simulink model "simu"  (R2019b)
settings: Solver=VariableStepAuto  StartTime=0.0  StopTime=10.0  RelTol=1e-3
libraries: fl_lib x81, nesl_utility x12

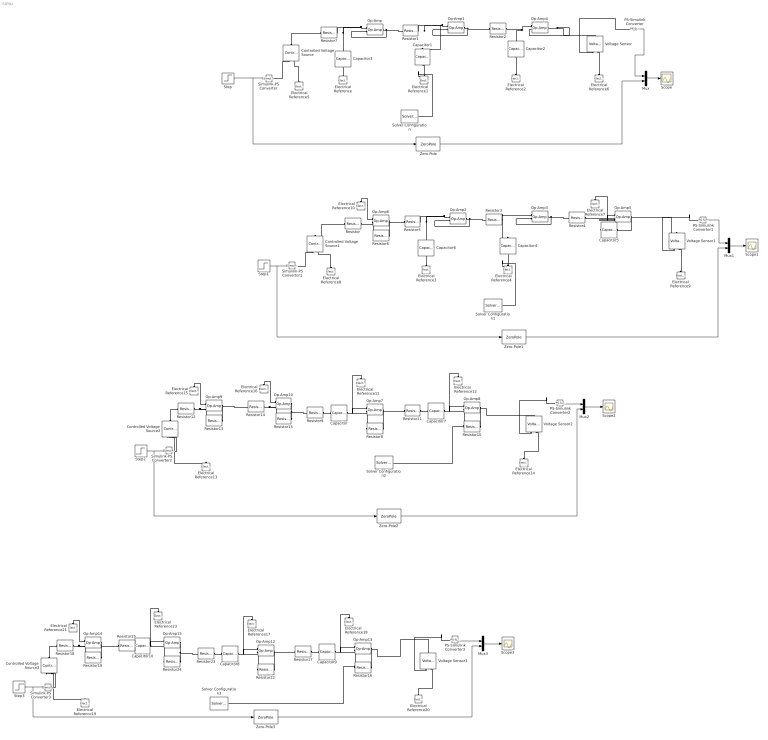
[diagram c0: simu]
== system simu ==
  Capacitor{,5,7..10} (6 alike) : fl_lib/Electrical/Electrical Elements/Capacitor  c=1 F  r=0 Ohm  g=0 1/Ohm  i_specify=off  i_priority=None  i=0 A  i_nominal_specify=off  i_nominal_unit=A  i_nominal_value=1  v_specify=off  v_priority=None  v=0 V  v_nominal_specify=off  v_nominal_unit=V  v_nominal_value=1  vc_specify=off  vc_priority=High  vc=0 V  vc_nominal_specify=off  vc_nominal_unit=V  vc_nominal_value=1
  Capacitor1 : fl_lib/Electrical/Electrical Elements/Capacitor  c=1/4 F  r=0 Ohm  g=0 1/Ohm  i_specify=off  i_priority=None  i=0 A  i_nominal_specify=off  i_nominal_unit=A  i_nominal_value=1  v_specify=off  v_priority=None  v=0 V  v_nominal_specify=off  v_nominal_unit=V  v_nominal_value=1  vc_specify=off  vc_priority=High  vc=0 V  vc_nominal_specify=off  vc_nominal_unit=V  vc_nominal_value=1
  Capacitor2 : fl_lib/Electrical/Electrical Elements/Capacitor  c=1/9 F  r=0 Ohm  g=0 1/Ohm  i_specify=off  i_priority=None  i=0 A  i_nominal_specify=off  i_nominal_unit=A  i_nominal_value=1  v_specify=off  v_priority=None  v=0 V  v_nominal_specify=off  v_nominal_unit=V  v_nominal_value=1  vc_specify=off  vc_priority=High  vc=0 V  vc_nominal_specify=off  vc_nominal_unit=V  vc_nominal_value=1
  Capacitor3 : fl_lib/Electrical/Electrical Elements/Capacitor  c=1/7 F  r=0 Ohm  g=0 1/Ohm  i_specify=off  i_priority=None  i=0 A  i_nominal_specify=off  i_nominal_unit=A  i_nominal_value=1  v_specify=off  v_priority=None  v=0 V  v_nominal_specify=off  v_nominal_unit=V  v_nominal_value=1  vc_specify=off  vc_priority=High  vc=0 V  vc_nominal_specify=off  vc_nominal_unit=V  vc_nominal_value=1
  Capacitor4 : fl_lib/Electrical/Electrical Elements/Capacitor  c=1/5 F  r=0 Ohm  g=0 1/Ohm  i_specify=off  i_priority=None  i=0 A  i_nominal_specify=off  i_nominal_unit=A  i_nominal_value=1  v_specify=off  v_priority=None  v=0 V  v_nominal_specify=off  v_nominal_unit=V  v_nominal_value=1  vc_specify=off  vc_priority=High  vc=0 V  vc_nominal_specify=off  vc_nominal_unit=V  vc_nominal_value=1
  Capacitor6 : fl_lib/Electrical/Electrical Elements/Capacitor  c=1/10 F  r=0 Ohm  g=0 1/Ohm  i_specify=off  i_priority=None  i=0 A  i_nominal_specify=off  i_nominal_unit=A  i_nominal_value=1  v_specify=off  v_priority=None  v=0 V  v_nominal_specify=off  v_nominal_unit=V  v_nominal_value=1  vc_specify=off  vc_priority=High  vc=0 V  vc_nominal_specify=off  vc_nominal_unit=V  vc_nominal_value=1
  Controlled Voltage Source{,1..3} (4 alike) : fl_lib/Electrical/Electrical Sources/Controlled Voltage Source
  Electrical Reference{,1..21,23} (23 alike) : fl_lib/Electrical/Electrical Elements/Electrical Reference
  Mux{,1..3} (4 alike) : Mux  Inputs=2
  Op-Amp{,1..10,12..15} (15 alike) : fl_lib/Electrical/Electrical Elements/Op-Amp  outI_specify=off  outI_priority=None  outI=0 A  outI_nominal_specify=off  outI_nominal_unit=A  outI_nominal_value=1
  PS-Simulink Converter{,1..3} (4 alike) : nesl_utility/PS-Simulink Converter  PhysicalDomain=network_engine_domain  SubClassName=ps_output  LeftPortType=input  RightPortType=output  PseudoPeriodic=off  Frequencies=[]  Unit=inherit  AffineConversion=off
  Resistor : fl_lib/Electrical/Electrical Elements/Resistor  R=150 Ohm  i_specify=off  i_priority=None  i=0 A  i_nominal_specify=off  i_nominal_unit=A  i_nominal_value=1  v_specify=off  v_priority=None  v=0 V  v_nominal_specify=off  v_nominal_unit=V  v_nominal_value=1
  Resistor{1..5,7..8,10..11,14..16,22,24} (14 alike) : fl_lib/Electrical/Electrical Elements/Resistor  R=1 Ohm  i_specify=off  i_priority=None  i=0 A  i_nominal_specify=off  i_nominal_unit=A  i_nominal_value=1  v_specify=off  v_priority=None  v=0 V  v_nominal_specify=off  v_nominal_unit=V  v_nominal_value=1
  Resistor12 : fl_lib/Electrical/Electrical Elements/Resistor  R=6 Ohm  i_specify=off  i_priority=None  i=0 A  i_nominal_specify=off  i_nominal_unit=A  i_nominal_value=1  v_specify=off  v_priority=None  v=0 V  v_nominal_specify=off  v_nominal_unit=V  v_nominal_value=1
  Resistor13 : fl_lib/Electrical/Electrical Elements/Resistor  R=3 Ohm  i_specify=off  i_priority=None  i=0 A  i_nominal_specify=off  i_nominal_unit=A  i_nominal_value=1  v_specify=off  v_priority=None  v=0 V  v_nominal_specify=off  v_nominal_unit=V  v_nominal_value=1
  Resistor17 : fl_lib/Electrical/Electrical Elements/Resistor  R=1/8 Ohm  i_specify=off  i_priority=None  i=0 A  i_nominal_specify=off  i_nominal_unit=A  i_nominal_value=1  v_specify=off  v_priority=None  v=0 V  v_nominal_specify=off  v_nominal_unit=V  v_nominal_value=1
  Resistor18 : fl_lib/Electrical/Electrical Elements/Resistor  R=1600 Ohm  i_specify=off  i_priority=None  i=0 A  i_nominal_specify=off  i_nominal_unit=A  i_nominal_value=1  v_specify=off  v_priority=None  v=0 V  v_nominal_specify=off  v_nominal_unit=V  v_nominal_value=1
  Resistor19 : fl_lib/Electrical/Electrical Elements/Resistor  R=4 Ohm  i_specify=off  i_priority=None  i=0 A  i_nominal_specify=off  i_nominal_unit=A  i_nominal_value=1  v_specify=off  v_priority=None  v=0 V  v_nominal_specify=off  v_nominal_unit=V  v_nominal_value=1
  Resistor23 : fl_lib/Electrical/Electrical Elements/Resistor  R=1/2 Ohm  i_specify=off  i_priority=None  i=0 A  i_nominal_specify=off  i_nominal_unit=A  i_nominal_value=1  v_specify=off  v_priority=None  v=0 V  v_nominal_specify=off  v_nominal_unit=V  v_nominal_value=1
  Resistor25 : fl_lib/Electrical/Electrical Elements/Resistor  R=1/100 Ohm  i_specify=off  i_priority=None  i=0 A  i_nominal_specify=off  i_nominal_unit=A  i_nominal_value=1  v_specify=off  v_priority=None  v=0 V  v_nominal_specify=off  v_nominal_unit=V  v_nominal_value=1
  Resistor6 : fl_lib/Electrical/Electrical Elements/Resistor  R=8 Ohm  i_specify=off  i_priority=None  i=0 A  i_nominal_specify=off  i_nominal_unit=A  i_nominal_value=1  v_specify=off  v_priority=None  v=0 V  v_nominal_specify=off  v_nominal_unit=V  v_nominal_value=1
  Resistor9 : fl_lib/Electrical/Electrical Elements/Resistor  R=1/6 Ohm  i_specify=off  i_priority=None  i=0 A  i_nominal_specify=off  i_nominal_unit=A  i_nominal_value=1  v_specify=off  v_priority=None  v=0 V  v_nominal_specify=off  v_nominal_unit=V  v_nominal_value=1
  Scope{,1..3} (4 alike) : Scope
  Simulink-PS Converter{,1..3} (4 alike) : nesl_utility/Simulink-PS Converter  PhysicalDomain=network_engine_domain  SubClassName=ps_input  LeftPortType=input  RightPortType=output  PseudoPeriodic=off  Frequencies=[]  NoiseDistribution=none  NoiseParameters=[]  Unit=1  AffineConversion=off  FilteringAndDerivatives=provide  SimscapeFilterOrder=1  InputFilterTimeConstant=0.001  UdotUserProvided=0
  Solver Configuration{,1..3} (4 alike) : nesl_utility/Solver Configuration  PhysicalDomain=network_engine_domain  SubClassName=solver  LeftPortType=input  RightPortType=generic  Tones=[]  Harmonics=[]  SimulateNoise=off  Profile=off  UseLocalSampling=off  EnableSwitchedLinearOptims=on  FrequencyDomain=off  UseCCode=off  RelTol=0.001  AbsTol=1e-06  MinStep=1e-09  ToWorkspace=off  RevertToSquareIcSolve=off  NumHomotopyIterations=100  PhasorMode=off  PhasorModeNumHarmonics=1  DoDC=off  ResidualTolerance=1e-09  UseLocalSolver=off  LocalSolverChoice=NE_BACKWARD_EULER_ADVANCER  LocalSolverSampleTime=0.001  DoFixedCost=off  MaxNonlinIter=3  MaxModeIter=2  LinearAlgebra=auto  EquationFormulation=NE_TIME_EF  DelaysMemoryBudget=1024  AutomaticFiltering=on  FilteringTimeConstant=0.001  PartitionStorageMethod=AS_NEEDED  PartitionMemoryBudget=1024  PartitionMethod=ROBUST
  Step{,1..3} (4 alike) : Step  SampleTime=0
  Voltage Sensor{,1..3} (4 alike) : fl_lib/Electrical/Electrical Sensors/Voltage Sensor
  Zero-Pole : ZeroPole  Zeros=[]  Poles=[-4 -7 -9]  Gain=[252]
  Zero-Pole1 : ZeroPole  Zeros=[]  Poles=[0 -10 -5]  Gain=[8/3]
  Zero-Pole2 : ZeroPole  Zeros=[0 0]  Poles=[-1 -6]  Gain=[3]
  Zero-Pole3 : ZeroPole  Zeros=[0 0 0]  Poles=[-2 -8 -.01]  Gain=[400/16]
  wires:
  Step/1 -> Zero-Pole/1, Simulink-PS Converter/1
  Mux/1 -> Scope/1
  Zero-Pole/1 -> Mux/2
  PS-Simulink Converter1/1 -> Mux1/1
  Mux1/1 -> Scope1/1
  Zero-Pole1/1 -> Mux1/2
  Step1/1 -> Zero-Pole1/1, Simulink-PS Converter1/1
  Step2/1 -> Zero-Pole2/1, Simulink-PS Converter2/1
  Mux2/1 -> Scope2/1
  PS-Simulink Converter2/1 -> Mux2/1
  Zero-Pole2/1 -> Mux2/2
  PS-Simulink Converter3/1 -> Mux3/1
  Mux3/1 -> Scope3/1
  Step3/1 -> Zero-Pole3/1, Simulink-PS Converter3/1
  Zero-Pole3/1 -> Mux3/2
  PS-Simulink Converter/1 -> Mux/1
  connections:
  Electrical Reference/LConn1 -- Capacitor3/LConn1
  Op-Amp/LConn1 -- Capacitor3/RConn1 -- Resistor7/RConn1
  Op-Amp/RConn1 -- Resistor1/LConn1 -- Op-Amp/LConn2
  Op-Amp1/LConn1 -- Capacitor1/RConn1 -- Resistor1/RConn1
  Electrical Reference1/LConn1 -- Capacitor1/LConn1 -- Solver Configuration/RConn1
  Op-Amp1/RConn1 -- Resistor2/LConn1 -- Op-Amp1/LConn2
  Op-Amp4/LConn1 -- Capacitor2/RConn1 -- Resistor2/RConn1
  Capacitor2/LConn1 -- Electrical Reference2/LConn1
  Op-Amp4/RConn1 -- Op-Amp4/LConn2 -- Voltage Sensor/LConn1
  Controlled Voltage Source/LConn1 -- Resistor7/LConn1
  Controlled Voltage Source/RConn2 -- Electrical Reference5/LConn1
  Simulink-PS Converter/RConn1 -- Controlled Voltage Source/RConn1
  Electrical Reference6/LConn1 -- Voltage Sensor/RConn2
  Voltage Sensor/RConn1 -- PS-Simulink Converter/LConn1
  Resistor3/RConn1 -- Op-Amp3/LConn1 -- Capacitor4/RConn1
  Op-Amp2/RConn1 -- Resistor3/LConn1 -- Op-Amp2/LConn2
  Electrical Reference4/LConn1 -- Capacitor4/LConn1 -- Solver Configuration1/RConn1
  Capacitor5/RConn1 -- Resistor4/RConn1 -- Op-Amp5/LConn2
  Op-Amp5/RConn1 -- Capacitor5/LConn1 -- Voltage Sensor1/LConn1
  Op-Amp3/RConn1 -- Resistor4/LConn1 -- Op-Amp3/LConn2
  Op-Amp2/LConn1 -- Capacitor6/RConn1 -- Resistor5/RConn1
  Voltage Sensor1/RConn1 -- PS-Simulink Converter1/LConn1
  Electrical Reference9/LConn1 -- Voltage Sensor1/RConn2
  Simulink-PS Converter1/RConn1 -- Controlled Voltage Source1/RConn1
  Controlled Voltage Source1/RConn2 -- Electrical Reference8/LConn1
  Electrical Reference3/LConn1 -- Capacitor6/LConn1
  Electrical Reference7/LConn1 -- Op-Amp5/LConn1
  Op-Amp6/RConn1 -- Resistor6/RConn1 -- Resistor5/LConn1
  Op-Amp6/LConn2 -- Resistor6/LConn1 -- Resistor/RConn1
  Resistor/LConn1 -- Controlled Voltage Source1/LConn1
  Electrical Reference10/LConn1 -- Op-Amp6/LConn1
  Op-Amp7/RConn1 -- Resistor11/LConn1 -- Resistor8/RConn1
  Op-Amp7/LConn2 -- Capacitor/RConn1 -- Resistor8/LConn1
  Capacitor/LConn1 -- Resistor9/RConn1
  Electrical Reference11/LConn1 -- Op-Amp7/LConn1
  Op-Amp8/LConn2 -- Capacitor7/RConn1 -- Solver Configuration2/RConn1 -- Resistor10/LConn1
  Electrical Reference12/LConn1 -- Op-Amp8/LConn1
  Capacitor7/LConn1 -- Resistor11/RConn1
  Op-Amp8/RConn1 -- Voltage Sensor2/LConn1 -- Resistor10/RConn1
  Electrical Reference13/LConn1 -- Controlled Voltage Source2/RConn2
  Simulink-PS Converter2/RConn1 -- Controlled Voltage Source2/RConn1
  Voltage Sensor2/RConn1 -- PS-Simulink Converter2/LConn1
  Electrical Reference14/LConn1 -- Voltage Sensor2/RConn2
  Resistor12/RConn1 -- Resistor13/LConn1 -- Op-Amp9/LConn2
  Op-Amp9/RConn1 -- Resistor13/RConn1 -- Resistor14/LConn1
  Electrical Reference15/LConn1 -- Op-Amp9/LConn1
  Controlled Voltage Source2/LConn1 -- Resistor12/LConn1
  Resistor14/RConn1 -- Resistor15/LConn1 -- Op-Amp10/LConn2
  Op-Amp10/RConn1 -- Resistor9/LConn1 -- Resistor15/RConn1
  Electrical Reference16/LConn1 -- Op-Amp10/LConn1
  Op-Amp14/RConn1 -- Resistor25/LConn1 -- Resistor19/RConn1
  Op-Amp13/RConn1 -- Voltage Sensor3/LConn1 -- Resistor16/RConn1
  Op-Amp13/LConn2 -- Capacitor9/RConn1 -- Solver Configuration3/RConn1 -- Resistor16/LConn1
  Resistor18/RConn1 -- Resistor19/LConn1 -- Op-Amp14/LConn2
  Op-Amp12/LConn2 -- Capacitor8/RConn1 -- Resistor22/LConn1
  Op-Amp12/RConn1 -- Resistor17/LConn1 -- Resistor22/RConn1
  Electrical Reference17/LConn1 -- Op-Amp12/LConn1
  Electrical Reference21/LConn1 -- Op-Amp14/LConn1
  Electrical Reference19/LConn1 -- Controlled Voltage Source3/RConn2
  Voltage Sensor3/RConn1 -- PS-Simulink Converter3/LConn1
  Controlled Voltage Source3/LConn1 -- Resistor18/LConn1
  Electrical Reference20/LConn1 -- Voltage Sensor3/RConn2
  Simulink-PS Converter3/RConn1 -- Controlled Voltage Source3/RConn1
  Capacitor8/LConn1 -- Resistor23/RConn1
  Capacitor9/LConn1 -- Resistor17/RConn1
  Electrical Reference18/LConn1 -- Op-Amp13/LConn1
  Op-Amp15/RConn1 -- Resistor24/RConn1 -- Resistor23/LConn1
  Op-Amp15/LConn2 -- Capacitor10/RConn1 -- Resistor24/LConn1
  Electrical Reference23/LConn1 -- Op-Amp15/LConn1
  Capacitor10/LConn1 -- Resistor25/RConn1
